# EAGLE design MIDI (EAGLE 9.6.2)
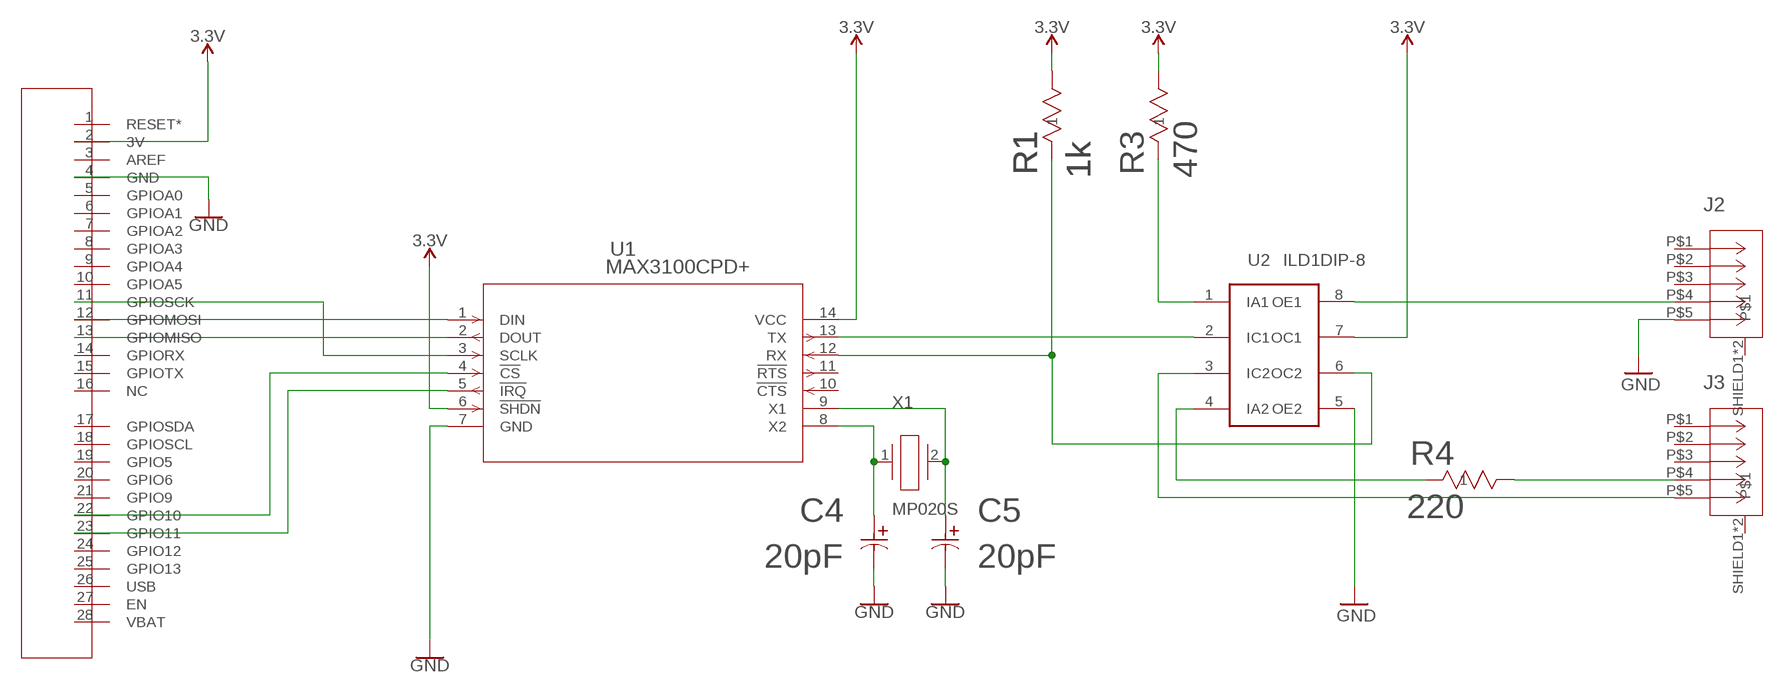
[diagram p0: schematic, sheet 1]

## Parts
C4  20pF  C317C200J5G5TA  [CAP_C317_KEM]
C5  20pF  C317C200J5G5TA  [CAP_C317_KEM]
J1  NRF52832_HEADER  [NRF52832_HEADER]
J2  5212044-1  [5212044]
J3  5212044-1  [5212044]
R1  1k  CF18JT47R0  [STA_CF18_STP]
R3  470  CF18JT220R  [STA_CF18_STP]
R4  220  CF18JT220R  [STA_CF18_STP]
U1  MAX3100CPD+  [21-0043D_14_MXM]
U2  ILD1DIP-8  [ILD1]
X1  MP020S  [CTS_MP]

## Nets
3.3V [supply]: J1.2(3V) R1.2 R3.2 U1.6(!SHDN) U1.14(VCC) U2.7(OC1)
GND [supply]: C4.2 C5.2 J1.4(GND) J2.P$5 U1.7(GND) U2.5(OE2)
N$1: U1.13(TX) U2.2(IC1)
N$2: J1.22(GPIO10) U1.4(!CS)
N$3: J1.23(GPIO11) U1.5(!IRQ)
N$4: J1.13(GPIOMISO) U1.2(DOUT)
N$5: J2.P$4 U2.8(OE1)
N$6: J1.12(GPIOMOSI) U1.1(DIN)
N$7: J1.11(GPIOSCK) U1.3(SCLK)
N$8: R3.1 U2.1(IA1)
N$9 [MIDI]: R4.1 U2.4(IA2)
N$10: C4.1 U1.8(X2) X1.1
N$12: C5.1 U1.9(X1) X1.2
N$13: R1.1 U1.12(RX) U2.6(OC2)
N$14 [MIDI]: J3.P$4 R4.2
N$17 [MIDI]: J3.P$5 U2.3(IC2)
Unconnected: J1.1(RESET*) J1.3(AREF) J1.5(GPIOA0) J1.6(GPIOA1) J1.7(GPIOA2) J1.8(GPIOA3) J1.9(GPIOA4) J1.10(GPIOA5) J1.14(GPIORX) J1.15(GPIOTX) J1.16(NC) J1.17(GPIOSDA) J1.18(GPIOSCL) J1.19(GPIO5) J1.20(GPIO6) J1.21(GPIO9) J1.24(GPIO12) J1.25(GPIO13) J1.26(USB) J1.27(EN) J1.28(VBAT) J2.P$1 J2.P$2 J2.P$3 J2.SHIELD1 J2.SHIELD2 J3.P$1 J3.P$2 J3.P$3 J3.SHIELD1 J3.SHIELD2 U1.10(!CTS) U1.11(!RTS)

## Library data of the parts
C4 C5 = Ben:C317C200J5G5TA
J1 = Ben:NRF52832_HEADER
J2 J3 = Ben:5212044-1
R1 = Ben:CF18JT47R0; BUILT_BY: EMA_UL_Team; MANUFACTURER_PART_NUMBER: CF18JT47R0; SOURCELIBRARY: Stackpole_2014-12-31; VENDOR: Stackpole International
R3 R4 = Ben:CF18JT220R; BUILT_BY: EMA_UL_Team; MANUFACTURER_PART_NUMBER: CF18JT220R; SOURCELIBRARY: Stackpole_2014-12-31; VENDOR: Stackpole International
U1 = maxim3100:MAX3100CPD+; BUILT_BY: EMA_UL_Team; MANUFACTURER_PART_NUMBER: max3100cpd+; SOURCELIBRARY: Maxim_2009-12-17_2; VENDOR: Maxim Integrated Products
U2 = Ben:ILD1: Vishay Semiconductors Optocoupler, Phototransistor Output (Dual Channel)
X1 = Ben:MP020S

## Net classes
0 default: width 0.254 mm
1 supply: width 0.61 mm, clearance 0.254 mm
2 MIDI: width 0.61 mm

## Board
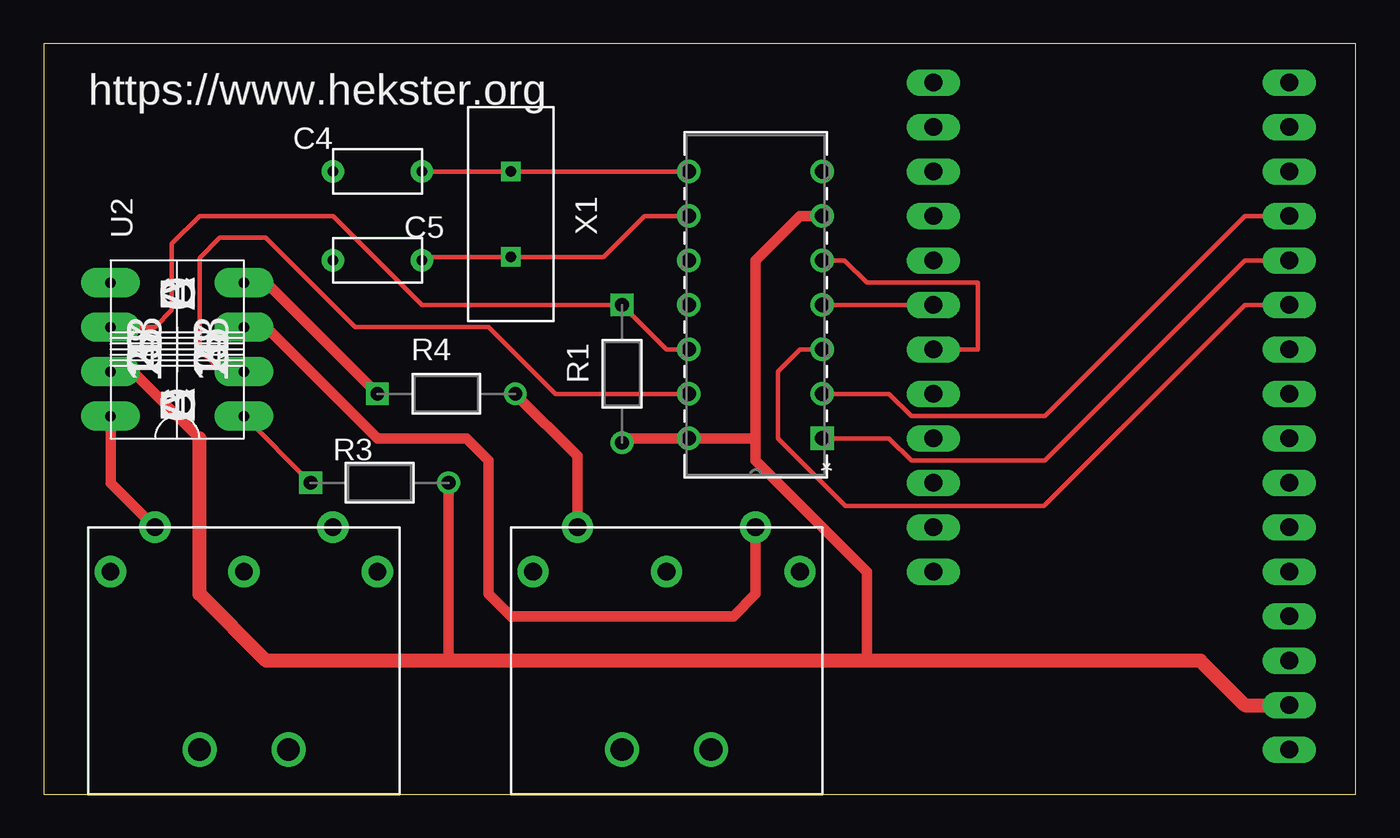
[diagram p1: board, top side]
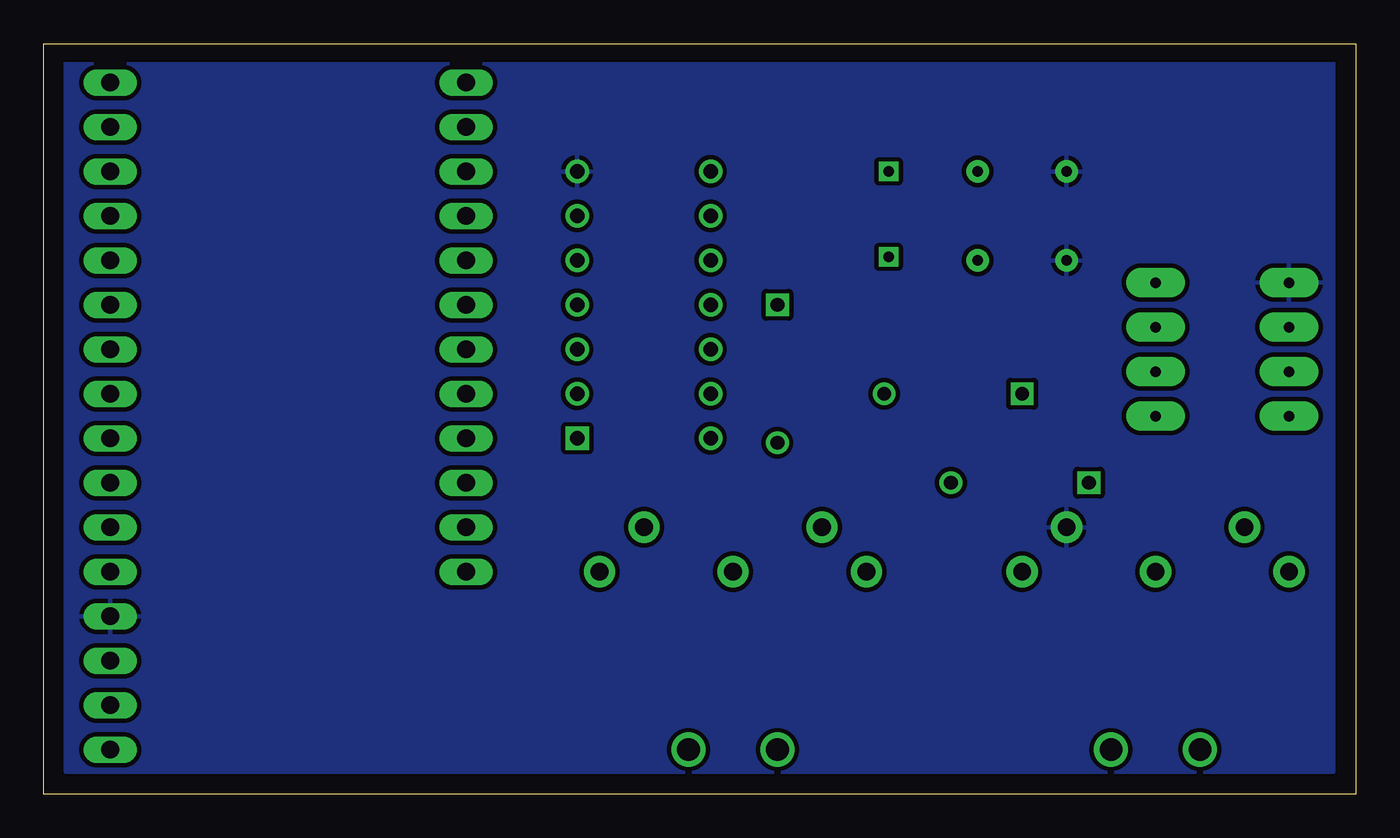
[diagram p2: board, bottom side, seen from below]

Size 74.91 x 42.85 mm. Coordinates in mm from the lower left corner, seen from the top.
Outline: 0,0 74.91,0 74.91,42.85 0,42.85 0,0
Copper layers (1*16): Top 0.035mm / dielectric 1.5mm / Bottom 0.035mm
Design rules "default": minimum track width 6mil, minimum drill 0.35mm, track to track 6mil, track to pad 6mil, pad to pad 6mil, via to via 6mil, smd to smd 6mil, copper to edge 40mil, drill to drill 6mil, minimum pad ring 10mil, minimum via ring 8mil, stop-mask expansion 4mil, vias tented up to drill 0mil, thermal gap 10mil

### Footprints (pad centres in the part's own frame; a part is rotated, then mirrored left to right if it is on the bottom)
CAP_C317_KEM = drill 0.6 pad 1.27: 1 0,0; 2 5.08,0
NRF52832_HEADER = drill 1.016 long: 1 0,0; 2 2.54,0; 3 5.08,0; 4 7.62,0; 5 10.16,0; 6 12.7,0; 7 15.24,0; 8 17.78,0; 9 20.32,0; 10 22.86,0; 11 25.4,0; 12 27.94,0; 13 30.48,0; 14 33.02,0; 15 35.56,0; 16 38.1,0; 17 38.1,20.32; 18 35.56,20.32; 19 33.02,20.32; 20 30.48,20.32; 21 27.94,20.32; 22 25.4,20.32; 23 22.86,20.32; 24 20.32,20.32; 25 17.78,20.32; 26 15.24,20.32; 27 12.7,20.32; 28 10.16,20.32
5212044 = drill 1.016 pad 1.778: P$1 15.24,2.54; P$2 7.62,2.54; P$3 0,2.54; P$4 12.7,0; P$5 2.54,0 | drill 1.295 pad 1.93: SHIELD1 10.16,12.7; SHIELD2 5.08,12.7
STA_CF18_STP = drill 0.787 pad 1.295 square: 1 0,0 | drill 0.787 pad 1.295: 2 7.874,0
21-0043D_14_MXM = drill 0.813 pad 1.321 square: 1 0,0 | drill 0.813 pad 1.321: 2 0,-2.54; 3 0,-5.08; 4 0,-7.62; 5 0,-10.16; 6 0,-12.7; 7 0,-15.24; 8 7.62,-15.24; 9 7.62,-12.7; 10 7.62,-10.16; 11 7.62,-7.62; 12 7.62,-5.08; 13 7.62,-2.54; 14 7.62,0
ILD1 = drill 0.6 pad 1.676 long: 1 0,-7.62; 2 2.54,-7.62; 3 5.08,-7.62; 4 7.62,-7.62; 5 7.62,0; 6 5.08,0; 7 2.54,0; 8 0,0
CTS_MP = drill 0.6 square: 1 0,0; 2 4.88,0

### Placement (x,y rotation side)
C4  21.59,35.56 180 top
C5  21.59,30.48 180 top
J1  71.12,2.54 90 top
J2  19.05,15.24 180 top
J3  43.18,15.24 180 top
R1  33.02,27.94 270 top
R3  15.24,17.78 0 top
R4  19.05,22.86 0 top
U1  44.45,20.32 180 top
U2  3.81,21.59 90 top
X1  26.67,35.56 270 top

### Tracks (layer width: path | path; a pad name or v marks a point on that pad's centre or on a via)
3.3V
  Top 0.61: U1.6 43.18,33.02 40.64,30.48 40.64,20.32 | 40.64,20.32 40.64,19.05 46.99,12.7 46.99,7.62 | 40.64,20.32 U1.14 33.27,20.32 R1.2 | 8.89,20.32 5.08,24.13 U2.7 | R3.2 23.11,7.62
  Top 0.813: J1.2 68.58,5.08 66.04,7.62 46.99,7.62 23.11,7.62 12.7,7.62 8.89,11.43 8.89,20.32
GND
  pour Bottom: 1.27,1.27 1.27,41.91 73.66,41.91 73.66,1.27
N$1
  Top 0.254: U1.13 29.21,22.86 25.4,26.67 17.78,26.67 12.67,31.78 10.06,31.78 8.89,30.61 8.89,25.4 10.16,24.13 U2.2
N$2
  Top 0.254: U1.4 J1.22
N$3
  Top 0.254: U1.5 45.72,30.48 46.99,29.21 53.34,29.21 53.34,25.4 J1.23
N$4
  Top 0.254: J1.13 68.58,33.02 57.15,21.59 49.53,21.59 48.26,22.86 U1.2
N$5
  Top 0.61: U2.8 3.81,17.78 J2.P$4
N$6
  Top 0.254: J1.12 68.58,30.48 57.15,19.05 49.53,19.05 48.26,20.32 U1.1
N$7
  Top 0.254: U1.3 43.18,25.4 41.91,24.13 41.91,20.32 45.77,16.46 57.1,16.46 68.58,27.94 J1.11
N$8
  Top 0.254: R3.1 U2.1
N$9
  Top 0.61: U2.4 12.7,29.21 R4.1
N$10
  Top 0.254: C4.1 X1.1 U1.8
N$12
  Top 0.254: U1.9 34.29,33.02 31.95,30.68 X1.2 21.79,30.68 C5.1
N$13
  Top 0.254: U1.12 35.56,25.4 R1.1 21.59,27.94 16.51,33.02 8.89,33.02 7.31,31.45 7.31,27.64 6.35,26.67 U2.6
N$14
  Top 0.61: J3.P$4 30.48,19.3 R4.2
N$17
  Top 0.61: J3.P$5 40.64,11.43 39.37,10.16 26.67,10.16 25.4,11.43 25.4,19.05 24.13,20.32 19.05,20.32 12.7,26.67 U2.3

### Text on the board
tPlace: https://www.hekster.org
